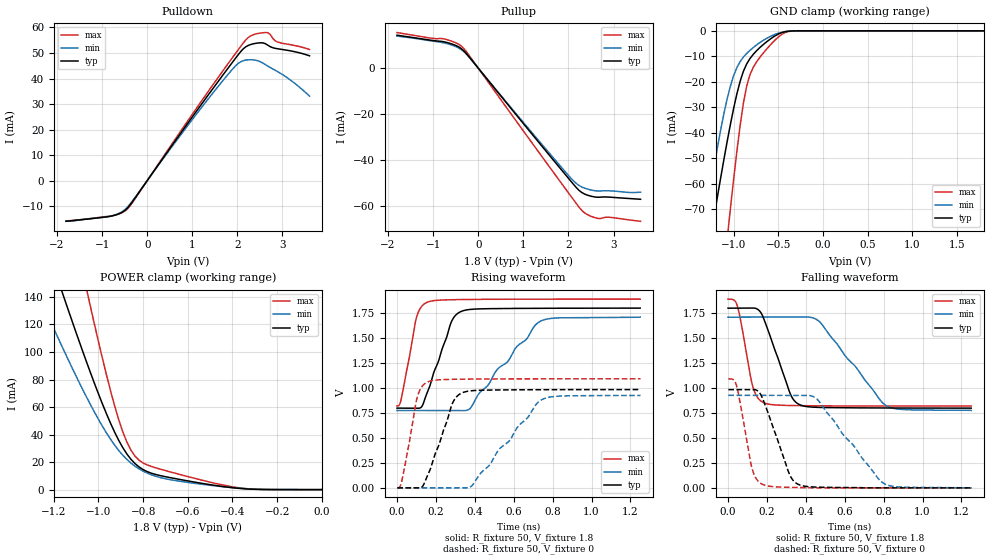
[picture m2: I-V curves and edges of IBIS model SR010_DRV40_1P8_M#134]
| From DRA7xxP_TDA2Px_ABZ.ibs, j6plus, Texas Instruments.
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| Model based on original model for DDR_DIFFIOPB_H
|   Sub model SR010_DRV40_1P8
[model]   SR010_DRV40_1P8_M#134
|[Description]  [1.8V-I/O-X-X]
|   , ,
|[Input Load]
|[Output Drive]
|Voltage   1.8V
|Mode   I/O
Model_type   I/O
Polarity   Non-Inverting
Enable   Active-Low
Vinl =  0.775
Vinh =  1.025
Cref =  15.0000pF
Rref =  100.0000M
Vref =  0V
Vmeas =  0.9
C_comp   2p   2p   2p
[Model Spec]
Vinl   0.78   0.735   0.825
Vinh   1.02   0.975   1.065
[Receiver Thresholds]
Tslew_ac = 0.5n
Vth = 0.9
Vth_max = 0.945
Vth_min = 0.81
Vinh_ac = 0.2
Vinh_dc = 0.125
Vinl_ac = -0.2
Vinl_dc = -0.125
[Temperature Range]   25   125   -40
[Voltage Range]   1.8   1.71   1.89
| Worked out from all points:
|   slope of the pulldown table from 0 to 0.27 V, typ, clamps not added: 39.7 ohm
|   slope of the pullup table from 0 to 0.27 V, typ, clamps not added: 41.4 ohm
|   GND clamp passes 1 mA (typ) near -0.48 V on its own axis
|   POWER clamp passes 1 mA (typ) near -0.38 V on its own axis
|   rising waveform, R_fixture 50, V_fixture 1.8: 20-80 % time 103ps typ, 248ps min, 59.7ps max; typ from 0.799 V to 1.8 V
|   rising waveform, R_fixture 50, V_fixture 0: 20-80 % time 101ps typ, 233ps min, 59.3ps max; typ from 0 V to 0.984 V
|   falling waveform, R_fixture 50, V_fixture 1.8: 20-80 % time 107ps typ, 227ps min, 59.9ps max; typ from 1.8 V to 0.799 V
|   falling waveform, R_fixture 50, V_fixture 0: 20-80 % time 105ps typ, 223ps min, 60ps max; typ from 0.984 V to 0 V
[POWER_clamp]
-1.8V     464.6mA    344.4mA    740.8mA
-1.273V   197mA      143.3mA    314.4mA
-1.164V   144mA      104.2mA    229mA
-1.145V   135.3mA    97.86mA    215mA
-1.055V   93.25mA    67.59mA    146.5mA
-1.036V   85.18mA    61.89mA    133.3mA
-909.1mV  35.72mA    28.41mA    50.73mA
-872.7mV  25.87mA    21.94mA    34.5mA
-818.2mV  16.45mA    15.08mA    21.33mA
-690.9mV  9.084mA    7.592mA    13.42mA
-400mV    1.38mA     1.43mA     2.039mA
0V        227.3nA    761nA      1.176uA
[Pulldown]
-1.8V     -15.9mA    -15.92mA   -15.81mA
-818.2mV  -13.96mA   -13.89mA   -13.92mA
-600mV    -12.8mA    -12.58mA   -12.84mA
-436.4mV  -10.71mA   -10.33mA   -11.03mA
1.255V    31.16mA    29.78mA    32.45mA
1.855V    45.52mA    42.91mA    47.32mA
2.073V    50.52mA    46.55mA    52.56mA
2.291V    53.3mA     47.36mA    56.66mA
2.618V    53.66mA    45.48mA    58mA
2.727V    52.47mA    44.31mA    57.26mA
2.891V    51.66mA    42.7mA     54.29mA
3.6V      48.88mA    33.12mA    51.37mA
[Pullup]
-1.8V     14.28mA    13.9mA     15.42mA
-1.036V   12.05mA    11.79mA    12.97mA
-763.6mV  11.43mA    10.95mA    12.69mA
-381.8mV  8.556mA    8.124mA    9.674mA
-218.2mV  5.258mA    5.122mA    5.967mA
2.018V    -48.25mA   -46.99mA   -54.63mA
2.182V    -52.02mA   -50.21mA   -58.98mA
2.291V    -53.95mA   -51.57mA   -61.66mA
2.455V    -55.39mA   -52.71mA   -63.95mA
2.673V    -56.09mA   -53.37mA   -65.34mA
2.891V    -56.02mA   -53.3mA    -64.76mA
3.6V      -56.97mA   -53.87mA   -66.53mA
[GND_clamp]
-1.8V     -200.8mA   -187.9mA   -345.9mA
-1.327V   -95.75mA   -76.22mA   -171.1mA
-1.255V   -80.19mA   -60.47mA   -144.9mA
-1.218V   -72.53mA   -52.92mA   -131.9mA
-1.073V   -43.32mA   -26.59mA   -81.54mA
-1.036V   -36.61mA   -21.6mA    -69.55mA
-963.6mV  -24.61mA   -14.37mA   -47.01mA
-854.5mV  -12.98mA   -8.864mA   -21.66mA
-781.8mV  -9.263mA   -6.573mA   -14.36mA
-672.7mV  -5.498mA   -3.827mA   -8.897mA
-345.5mV  -48.81uA   -73.08uA   -79.37uA
1.8V      227.3nA    3.986uA    988nA
[Ramp]
dV/dt_f 0.60153424/0.10744776n 0.56192781/0.2273118n 0.64277767/59.968497p
dV/dt_r 0.59177899/0.10139258n 0.55724385/0.23420596n  0.6561862/59.423309p
R_load = 50
[Rising Waveform]
R_fixture = 50
V_fixture = 1.8
V_fixture_min = 1.71
V_fixture_max = 1.89
0s        798.6mV    774.9mV    820.3mV
21.72ps   798.3mV    774.9mV    889.2mV
100.9ps   797.5mV    774.8mV    1.712V
128.2ps   816.2mV    774.8mV    1.821V
154.4ps   949.4mV    774.8mV    1.858V
278.8ps   1.659V     774.7mV    1.884V
332.6ps   1.769V     773.3mV    1.886V
377.3ps   1.787V     798.6mV    1.887V
736ps     1.798V     1.667V     1.89V
1.25ns    1.8V       1.71V      1.89V
[Rising Waveform]
R_fixture = 50
V_fixture = 0
V_fixture_min = 0
V_fixture_max = 0
1.859ps   0V         0V         0V
25.92ps   0V         0V         80.53mV
103.9ps   0V         0V         907.3mV
130.7ps   13.21mV    0V         1.021V
156.9ps   124.1mV    0V         1.06V
283.7ps   841mV      0V         1.087V
337.9ps   954.1mV    0V         1.089V
387.3ps   973.2mV    26.23mV    1.089V
746.3ps   983mV      885.5mV    1.092V
1.252ns   984.5mV    926.8mV    1.092V
[Falling Waveform]
R_fixture = 50
V_fixture = 1.8
V_fixture_min = 1.71
V_fixture_max = 1.89
0s        1.8V       1.71V      1.89V
46.21ps   1.8V       1.71V      1.833V
127.1ps   1.801V     1.71V      1.018V
150.6ps   1.791V     1.71V      907.8mV
184.6ps   1.69V      1.71V      852mV
320.6ps   939.7mV    1.71V      825.1mV
370ps     831.7mV    1.71V      823.5mV
472.5ps   805.6mV    1.66V      821.5mV
816.7ps   800.1mV    819.6mV    819.5mV
1.25ns    798.6mV    774.9mV    819.3mV
[Falling Waveform]
R_fixture = 50
V_fixture = 0
V_fixture_min = 0
V_fixture_max = 0
1.859ps   984.5mV    926.8mV    1.092V
41.81ps   984.7mV    926.8mV    1.035V
122.4ps   985mV      926.9mV    203.3mV
143.8ps   981mV      926.9mV    95.48mV
176.7ps   900.3mV    926.8mV    35.54mV
313.6ps   146.5mV    926.7mV    5.305mV
363.3ps   33.11mV    926.9mV    3.503mV
460.5ps   7.065mV    883mV      0V
804.2ps   0V         40.67mV    0V
1.252ns   0V         0V         0V
